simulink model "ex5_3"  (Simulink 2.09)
settings: Solver=ode45  StartTime=0.0  StopTime=40  RelTol=1e-3  AbsTol=1e-6

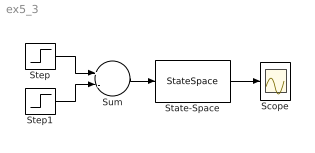
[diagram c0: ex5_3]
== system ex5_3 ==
  Scope : Scope
  State-Space : StateSpace  A=[0,1;-0.4,-0.2]  B=[0;0.2]  C=[1,0]  D=[0]  X0=[0;0]
  Step : Step  Time=0  Before=0  After=100
  Step1 : Step  Time=0.01  Before=0  After=100
  Sum : Sum  Inputs=+-
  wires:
  Step1/1 -> Sum/2
  State-Space/1 -> Scope/1
  Sum/1 -> State-Space/1
  Step/1 -> Sum/1
